ORGANIZATION_BLOCK OB 1
TITLE = "Main Program Sweep (Cycle)"
//1. Read/Write
//-------------
//
//This program is a simple example for reading the actual key-ID consistently by
//using SFC14.
//
//Use VAT_KP to see the ID and to set the LED control.
AUTHOR : RAmann
FAMILY : KP
NAME : KPMAIN
VERSION : 1.0


VAR_TEMP
  OB1_EV_CLASS : BYTE ;	//Bits 0-3 = 1 (Coming event), Bits 4-7 = 1 (Event class 1)
  OB1_SCAN_1 : BYTE ;	//1 (Cold restart scan 1 of OB 1), 3 (Scan 2-n of OB 1)
  OB1_PRIORITY : BYTE ;	//Priority of OB Execution
  OB1_OB_NUMBR : BYTE ;	//1 (Organization block 1, OB1)
  OB1_RESERVED_1 : BYTE ;	//Reserved for system
  OB1_RESERVED_2 : BYTE ;	//Reserved for system
  OB1_PREV_CYCLE : INT ;	//Cycle time of previous OB1 scan (milliseconds)
  OB1_MIN_CYCLE : INT ;	//Minimum cycle time of OB1 (milliseconds)
  OB1_MAX_CYCLE : INT ;	//Maximum cycle time of OB1 (milliseconds)
  OB1_DATE_TIME : DATE_AND_TIME ;	//Date and time OB1 started
END_VAR
BEGIN
NETWORK
TITLE =read actual key-ID

      CALL SFC   14 (
           LADDR                    := W#16#A,//input address 10 (Ah)
           RET_VAL                  := MW     2,//dummy
           RECORD                   := P#M 10.0 BYTE 8);//buffer for Key-ID (8 bytes from MB10 to MB17)

NETWORK
TITLE =LED control

      U     M     18.0;
      =     A     10.0; //LED red

      U     M     18.1;
      =     A     10.1; //LED green

END_ORGANIZATION_BLOCK

